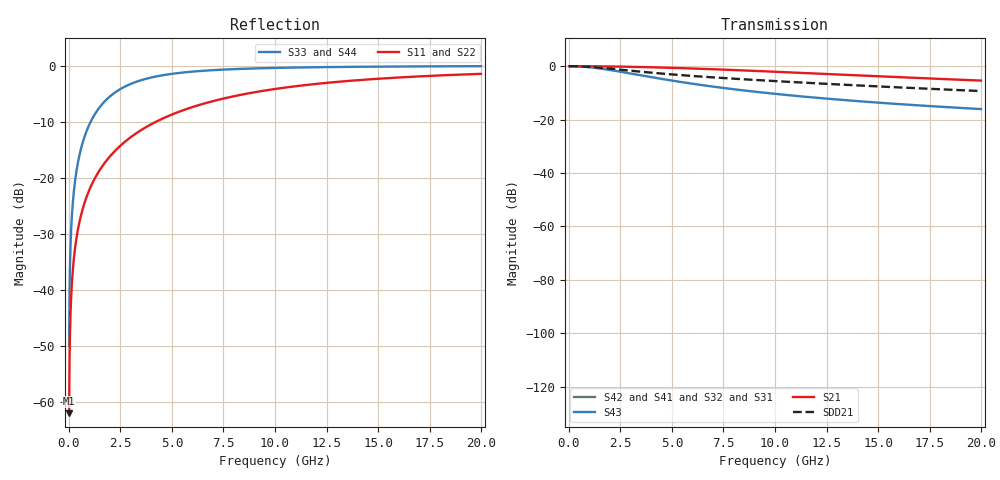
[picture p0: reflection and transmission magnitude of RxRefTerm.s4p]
! 0.5 pF port 1 to ground & 2 pF port 2 to ground  (Model #2 from T10/07-267r0)
! reasonably models 6G SAS high frequency limits for SDD11 & SCD11
!  Mike Jenkins  5 June 2007
# MHz S MA R 50
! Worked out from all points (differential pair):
!   1999 points, 10 MHz to 19.99 GHz, reference 50 ohm
!   strongest paths, dB at 10 MHz, 5 GHz, 10 GHz, 15 GHz, 19.99 GHz:
!     S21: 0.0, -0.6, -2.1, -3.8, -5.4
!     S43: 0.0, -5.4, -10.4, -13.7, -16.1
!     S42: -, -, -, -, -
!     S41: -, -, -, -, -
!     S32: -, -, -, -, -
!     S31: -, -, -, -, -
!   taken as a pair (ports 1,3 in; 2,4 out), SDD21 dB: 0.0, -3.1, -5.6, -7.6, -9.3
!   lowest |S11| = -62.1 dB at 10 MHz (marker M1), VSWR 1.00, Z = 50 - j0.0785 ohm
!   |S11| at or under -10 dB: start of sweep to 4.244 GHz
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10  0.000785 -90.0  1 -0.0  0 0.0  0 0.0
    1 -0.0  0.000785 -90.0  0 0.0  0 0.0
    0 0.0  0 0.0  0.003142 -90.2  1 -0.2
    0 0.0  0 0.0  1 -0.2  0.003142 -90.2
200  0.01571 -90.9  0.9999 -0.9  0 0.0  0 0.0
     0.9999 -0.9  0.01571 -90.9  0 0.0  0 0.0
     0 0.0  0 0.0  0.06271 -93.6  0.998 -3.6
     0 0.0  0 0.0  0.998 -3.6  0.06271 -93.6
640  0.0502 -92.9  0.9987 -2.9  0 0.0  0 0.0
     0.9987 -2.9  0.0502 -92.9  0 0.0  0 0.0
     0 0.0  0 0.0  0.1971 -101.4  0.9804 -11.4
     0 0.0  0 0.0  0.9804 -11.4  0.1971 -101.4
1550  0.1208 -96.9  0.9927 -6.9  0 0.0  0 0.0
      0.9927 -6.9  0.1208 -96.9  0 0.0  0 0.0
      0 0.0  0 0.0  0.4378 -116.0  0.8991 -26.0
      0 0.0  0 0.0  0.8991 -26.0  0.4378 -116.0
3060  0.2337 -103.5  0.9723 -13.5  0 0.0  0 0.0
      0.9723 -13.5  0.2337 -103.5  0 0.0  0 0.0
      0 0.0  0 0.0  0.693 -133.9  0.7209 -43.9
      0 0.0  0 0.0  0.7209 -43.9  0.693 -133.9
8040  0.5339 -122.3  0.8455 -32.3  0 0.0  0 0.0
      0.8455 -32.3  0.5339 -122.3  0 0.0  0 0.0
      0 0.0  0 0.0  0.9298 -158.4  0.3681 -68.4
      0 0.0  0 0.0  0.3681 -68.4  0.9298 -158.4
19990  0.8434 -147.5  0.5372 -57.5  0 0.0  0 0.0
       0.5372 -57.5  0.8434 -147.5  0 0.0  0 0.0
       0 0.0  0 0.0  0.9876 -170.9  0.1573 -81.0
       0 0.0  0 0.0  0.1573 -81.0  0.9876 -170.9
